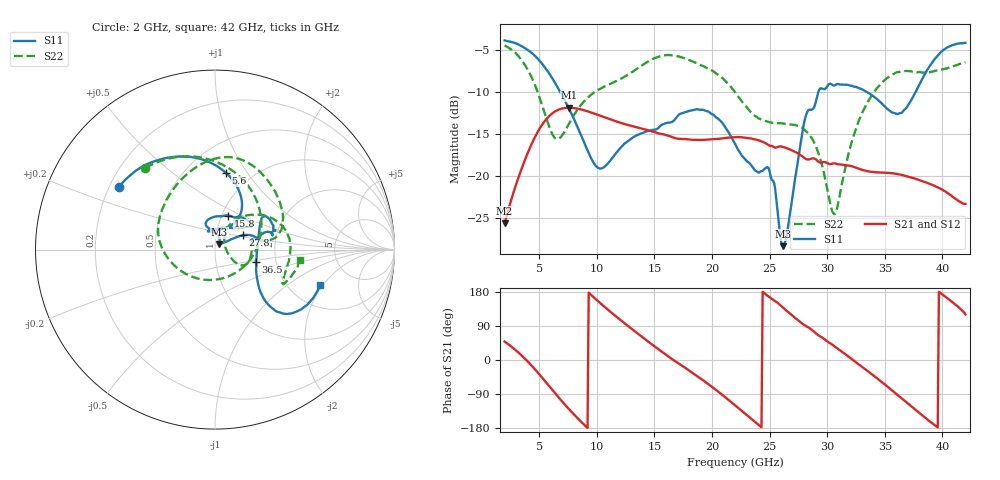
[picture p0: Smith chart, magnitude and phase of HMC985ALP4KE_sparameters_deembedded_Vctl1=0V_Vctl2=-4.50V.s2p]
!s2p File: Measurements: S11, S21, S12, S22
# GHz S dB R 50.0
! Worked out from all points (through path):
!   401 points, 2 GHz to 42 GHz, reference 50 ohm
!   highest |S21| = -11.90 dB at 7.6 GHz (marker M1); lowest = -25.7 dB at 2 GHz (marker M2)
!   lowest |S11| = -28.4 dB at 26.2 GHz (marker M3), VSWR 1.08, Z = 52.3 + j3.17 ohm
!   |S11| at or under -10 dB: 6.82 GHz to 29.25 GHz (22.43 GHz wide, 124 % of centre); 33.42 GHz to 37.69 GHz (4.269 GHz wide, 12 % of centre)
!   |S22| runs from -24.6 to -4.5 dB; largest |S21 - S12| = 0.00021
!   S11 on the Smith chart (normalised r, x): 2 GHz: 0.24, +0.28; 5.6 GHz: 0.76, +0.80; 15.8 GHz: 1.07, +0.42; 27.8 GHz: 1.34, +0.22; 36.5 GHz: 1.57, -0.23; 42 GHz: 2.94, -1.89
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2  -3.88 147.0  -25.66 48.6  -25.67 48.6  -4.47 130.5
3.6  -4.66 120.3  -18.70 8.4  -18.70 8.4  -6.47 84.9
4.7  -5.80 99.5  -15.22 -26.8  -15.22 -26.8  -9.42 43.4
5.6  -7.29 81.9  -13.29 -59.1  -13.30 -59.1  -13.05 -3.7
6.5  -9.22 66.5  -12.25 -92.0  -12.25 -92.0  -15.61 -68.9
7.6  -12.04 54.8  -11.90 -130.1  -11.90 -130.1  -13.77 -135.8
8.7  -15.38 55.1  -12.12 -164.7  -12.12 -164.7  -11.44 -170.2
10.4  -19.13 89.6  -12.89 147.5  -12.90 147.5  -9.56 162.4
15.4  -14.22 75.7  -14.97 27.5  -14.97 27.5  -5.80 87.1
15.8  -13.83 68.7  -15.07 18.6  -15.07 18.6  -5.67 82.0
19.4  -12.23 33.3  -15.72 -57.3  -15.72 -57.3  -7.05 35.0
22  -16.18 51.1  -15.40 -119.4  -15.41 -119.5  -10.05 9.9
24.9  -19.04 104.7  -16.34 167.9  -16.35 167.8  -13.58 13.2
26.2  -28.38 52.6  -16.58 137.4  -16.58 137.4  -13.78 -2.5
27.8  -15.22 27.2  -17.64 97.0  -17.64 96.9  -14.25 -24.4
28.7  -12.11 12.6  -17.93 78.8  -17.94 78.8  -15.58 -31.5
30.7  -9.21 20.8  -18.53 34.5  -18.54 34.5  -24.51 23.2
32.8  -9.59 33.9  -19.19 -13.1  -19.20 -13.1  -13.26 53.4
35.4  -12.22 11.8  -19.66 -74.3  -19.66 -74.3  -8.17 21.4
36.5  -12.47 -16.7  -19.90 -102.1  -19.91 -102.1  -7.54 7.3
39.5  -5.86 -43.8  -21.30 -175.5  -21.31 -175.6  -7.47 -26.3
42  -4.16 -18.6  -23.34 120.3  -23.35 120.3  -6.47 -7.2
